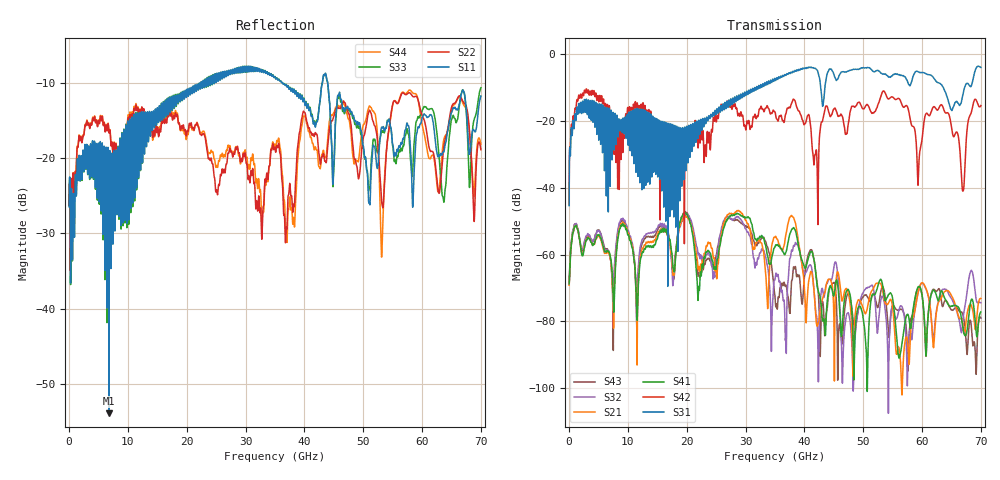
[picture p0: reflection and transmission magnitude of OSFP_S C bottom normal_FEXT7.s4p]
! AWR Design Environment (8415) Mon Jan 07 17:19:05 2019
! Document = 'OSFP Channel_S'
! nPorts: 4, nXvals: 7001
# HZ S DB R 50
!Freq DBS11 AngS11 DBS12 AngS12 DBS13 AngS13 DBS14 AngS14
!	DBS21 AngS21 DBS22 AngS22 DBS23 AngS23 DBS24 AngS24
!	DBS31 AngS31 DBS32 AngS32 DBS33 AngS33 DBS34 AngS34
!	DBS41 AngS41 DBS42 AngS42 DBS43 AngS43 DBS44 AngS44
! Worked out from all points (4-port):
!   7000 points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, 10 MHz to 70 GHz, reference 50 ohm
!   strongest paths, dB at 10 MHz, 17.51 GHz, 35.01 GHz, 52.51 GHz, 70 GHz:
!     S31: -45.4, -27.5, -7.4, -4.9, -4.0
!     S42: -45.1, -34.5, -17.4, -15.1, -15.4
!     S41: -68.8, -60.0, -57.7, -69.3, -77.2
!     S21: -69.2, -62.1, -54.7, -68.6, -73.1
!     S32: -68.4, -64.8, -67.2, -82.0, -74.4
!     S43: -67.2, -61.6, -72.6, -75.7, -79.0
!   lowest |S11| = -53.9 dB at 6.78 GHz (marker M1), VSWR 1.00, Z = 50.1 - j0.161 ohm
!   |S11| at or under -10 dB: start of sweep to 22.43 GHz; 36.26 GHz to 43.05 GHz (6.791 GHz wide, 17.1 % of centre); 43.96 GHz to end of sweep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
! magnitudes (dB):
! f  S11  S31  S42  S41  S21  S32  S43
! 10 MHz  -26.5  -45.4  -45.1  -68.8  -69.2  -68.4  -67.2
! 6.78 GHz  -53.9  -17.1  -16.0  -59.1  -59.6  -59.1  -59.0
! 37.87 GHz  -10.8  -5.7  -14.6  -52.4  -48.4  -58.7  -67.7
! 42.08 GHz  -15.2  -4.7  -29.4  -68.0  -80.9  -78.4  -67.3
! 53.49 GHz  -16.1  -5.9  -11.1  -71.8  -72.9  -73.6  -70.3
! 66.94 GHz  -11.0  -12.2  -41.0  -82.0  -80.9  -79.8  -78.0
! 70 GHz  -11.8  -4.0  -15.4  -77.2  -73.1  -74.4  -79.0
